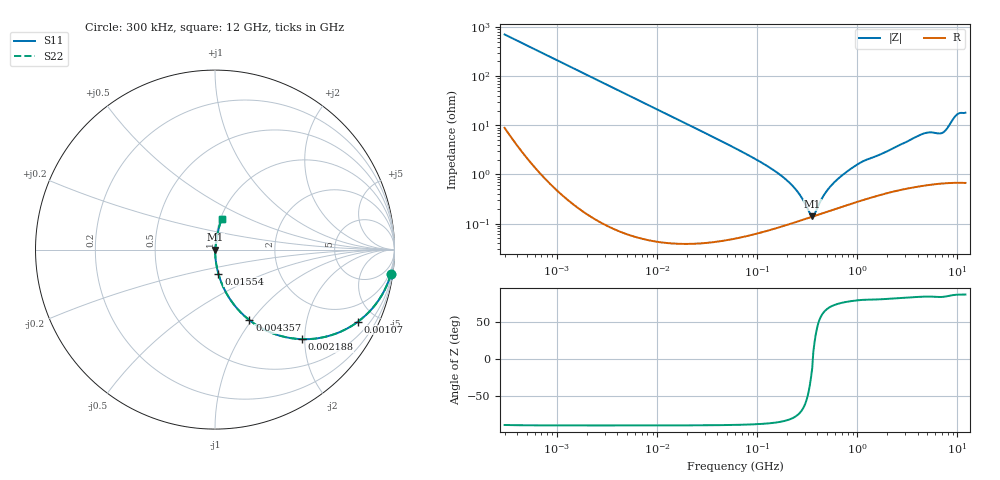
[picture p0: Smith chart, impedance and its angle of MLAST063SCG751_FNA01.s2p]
! MLAST063SCG751_FNA01  S-PARAMETER MODEL  ( General Type )
! Model Generated by TAIYO YUDEN Corporation (http://www.ty-top.com)
! Version 1.0
! TAIYO YUDEN Control No. 160830
! Copyright(c) 2016 TAIYO YUDEN CO.,LTD. All Rights Reserved.
! Product Description (link to TY-COMPAS)
! https://ds.yuden.co.jp/TYCOMPAS/or/detail?pn=MLAST063SCG751JFNA01&u=M
! Products Name : Multilayer Ceramic Capacitors
! Characteristics :
!  Capacitance : 750 pF , Rated Voltage : 25V , TCC : CG / C0G
!  Case Size : 0.6 x 0.3 / 0.024 x 0.012 [mm/inch] , Thickness : 0.3 / 0.012 [mm/inch]
!  (Conditions: Temperature = 25 degC , DC Bias Current/Voltage = 0A / 0V)
! External Node Assignments :
!  1  o---| |---o  2
! GND o---------o GND
! Frequency Range : 0.3MHz  -  12000MHz  [ 401 STEP ]
# MHz S RI R 50
! Freq[MHz].  S11 Real  S11 Imag  S21 Real  S21 Imag  S12 Real  S12 Imag  S22 Real  S22 Imag
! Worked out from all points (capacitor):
!   401 points, 300 kHz to 12 GHz, reference 50 ohm
!   read as one part in series: C = 750 pF near 316.3 kHz
!   lowest |Z| = 141 mohm at 354 MHz (marker M1)
!   series resonance near 359.2 MHz, so ESL is about 260 pH
!   S11 on the Smith chart (normalised r, x): 300 kHz: 1, -14; 1.07 MHz: 1.01, -3.97; 2.188 MHz: 1.00, -1.94; 4.357 MHz: 1.00, -0.97; 15.54 MHz: 1.00, -0.27; 12 GHz: 1.01, +0.36
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0.3  0.9787 -0.1381  0.0213 0.1381  0.0213 0.1381  0.9787 -0.1381
0.613423  0.922 -0.2662  0.078 0.2662  0.078 0.2662  0.922 -0.2662
1.069962  0.7968 -0.4013  0.2032 0.4013  0.2032 0.4013  0.7968 -0.4013
1.769972  0.5896 -0.4911  0.4104 0.4911  0.4104 0.4911  0.5896 -0.4911
2.187799  0.4848 -0.4991  0.5152 0.4991  0.5152 0.4991  0.4848 -0.4991
4.356537  0.1921 -0.3932  0.8079 0.3932  0.8079 0.3932  0.1921 -0.3932
10.44266  0.04 -0.1948  0.96 0.1948  0.96 0.1948  0.04 -0.1948
15.53777  0.0186 -0.1337  0.9814 0.1337  0.9814 0.1337  0.0186 -0.1337
60  0.00167 -0.0343  0.9983 0.0343  0.9983 0.0343  0.00167 -0.0343
122.6847  0.000936 -0.0153  0.9991 0.0153  0.9991 0.0153  0.000936 -0.0153
192.4766  0.000984 -0.00792  0.999 0.00792  0.999 0.00792  0.000984 -0.00792
257.5933  0.00113 -0.00409  0.9989 0.00409  0.9989 0.00409  0.00113 -0.00409
353.9943  0.00138 -0.000308  0.9986 0.000308  0.9986 0.000308  0.00138 -0.000308
373.2558  0.00143 0.000589  0.9986 -0.000589  0.9986 -0.000589  0.00143 0.000589
499.5319  0.00176 0.00438  0.9982 -0.00438  0.9982 -0.00438  0.00176 0.00438
668.5285  0.0022 0.00849  0.9978 -0.00849  0.9978 -0.00849  0.0022 0.00849
1105.905  0.00326 0.0177  0.9967 -0.0177  0.9967 -0.0177  0.00326 0.0177
2088.533  0.0052 0.0306  0.9948 -0.0306  0.9948 -0.0306  0.0052 0.0306
4623.766  0.0104 0.0672  0.9896 -0.0672  0.9896 -0.0672  0.0104 0.0672
7064.448  0.0113 0.0687  0.9887 -0.0687  0.9887 -0.0687  0.0113 0.0687
9708.23  0.0312 0.1541  0.9688 -0.1541  0.9688 -0.1541  0.0312 0.1541
12000  0.0376 0.1725  0.9624 -0.1725  0.9624 -0.1725  0.0376 0.1725
